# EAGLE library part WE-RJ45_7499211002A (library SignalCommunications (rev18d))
Order Code 7499211002A Design THT xBase-T 10/100 Base-T PoE Ports 1x1 Application PoE Tab Position DOWN LED (Left-Right) NONE EMI Fingers Yes Details see: http://katalog.we-online.de/en/pbs/WE-LAN_RJ45/7499211002A? Updated by Yingchun Shan 2016-08-30 2016(C) Würth Elektronik
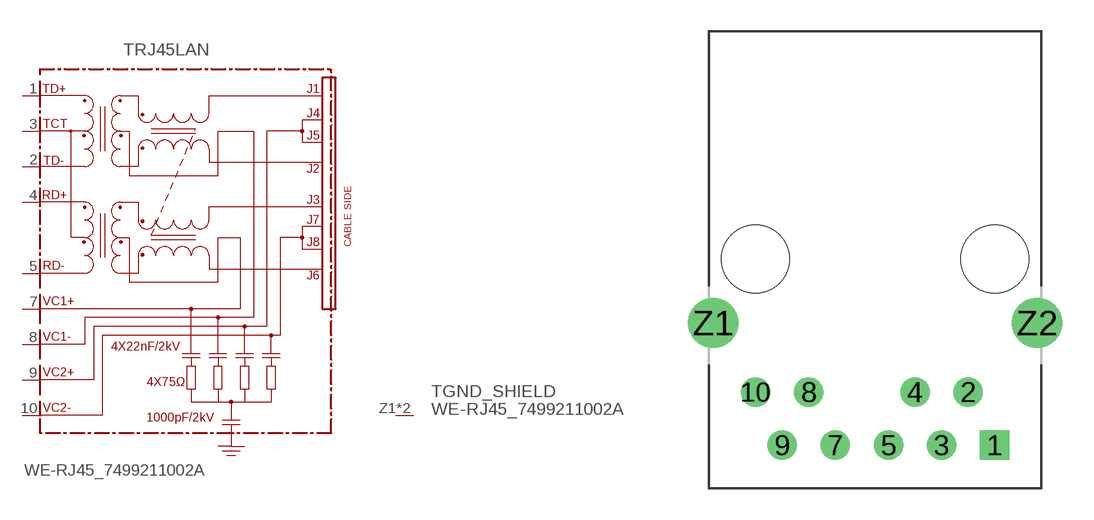
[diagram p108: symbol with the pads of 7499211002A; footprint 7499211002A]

Designator prefix T; gates RJ45LAN=749921-TYPE-2-RVS GND_SHIELD=GNDPIN

## WE-RJ45_7499211002A (COMPANY-URL: http://www.we-online.de; CREATED-BY: Christin Zierenner; CREATED-DATE: AUG 2012; DATASHEET-URL: http://katalog.we-online.de/kataloge/eisos/media/pdf/7499211002A.pdf; MANUFACTURER: Würth Elektronik eiSos GmbH)  [7499211002A]
1  RJ45LAN:TD+
2  RJ45LAN:TD-
3  RJ45LAN:TCT
4  RJ45LAN:RD+
5  RJ45LAN:RD-
7  RJ45LAN:VC1+  pwr
8  RJ45LAN:VC1-  pwr
9  RJ45LAN:VC2+  pwr
10  RJ45LAN:VC2-  pwr
Z1  GND_SHIELD:GND  pwr
Z2  GND_SHIELD:GND  pwr

## Footprint 7499211002A (pad centres in mm)
MAX HEIGHT=13.74mm PORTS----1X1 LED ----NO
drill 0.9 square: 1 5.715,-8.89
drill 0.9: 2 4.445,-6.35; 3 3.175,-8.89; 4 1.905,-6.35; 5 0.635,-8.89; 7 -1.905,-8.89; 8 -3.175,-6.35; 9 -4.445,-8.89; 10 -5.715,-6.35
drill 1.6: Z1 -7.74,-3.05; Z2 7.74,-3.05
hole 3.25 at 5.715,0
hole 3.25 at -5.715,0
